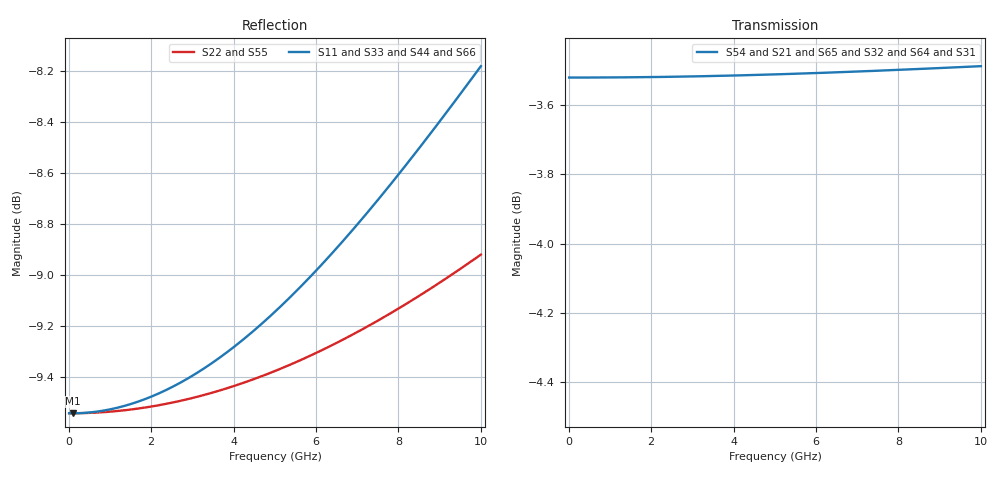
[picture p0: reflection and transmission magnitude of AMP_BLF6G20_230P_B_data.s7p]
! Created Tue Mar 30 08:44:35 2010
# ghz S ma R 50
! 7 Port Network Data from SP1.SP block
! freq  magS11  angS11  magS12  angS12  magS13  angS13  magS14  angS14
!  magS15  angS15  magS16  angS16  magS17  angS17
!  magS21  angS21
!  magS22  angS22  magS23  angS23  magS24  angS24  magS25  angS25
!  magS26  angS26  magS27  angS27
!  magS31  angS31  magS32  angS32
!  magS33  angS33  magS34  angS34  magS35  angS35  magS36  angS36
!  magS37  angS37
!  magS41  angS41  magS42  angS42  magS43  angS43
!  magS44  angS44  magS45  angS45  magS46  angS46  magS47  angS47
!  magS51  angS51  magS52  angS52  magS53  angS53  magS54  angS54
!  magS55  angS55  magS56  angS56  magS57  angS57
!  magS61  angS61
!  magS62  angS62  magS63  angS63  magS64  angS64  magS65  angS65
!  magS66  angS66  magS67  angS67
!  magS71  angS71  magS72  angS72
!  magS73  angS73  magS74  angS74  magS75  angS75  magS76  angS76
!  magS77  angS77
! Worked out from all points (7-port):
!   1000 points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, 10 MHz to 10 GHz, reference 50 ohm
!   strongest paths, dB at 10 MHz, 2.51 GHz, 5.01 GHz, 7.51 GHz, 10 GHz:
!     S54: -3.5, -3.5, -3.5, -3.5, -3.5
!     S21: -3.5, -3.5, -3.5, -3.5, -3.6
!     S65: -3.5, -3.5, -3.5, -3.6, -3.6
!     S32: -3.5, -3.5, -3.6, -3.6, -3.7
!     S64: -3.5, -3.5, -3.6, -3.7, -3.9
!     S31: -3.5, -3.5, -3.6, -3.7, -3.9
!   lowest |S11| = -9.5 dB at 100 MHz (marker M1), VSWR 2.00, Z = 25 + j0.174 ohm
!   |S11| at or under -10 dB: nowhere
